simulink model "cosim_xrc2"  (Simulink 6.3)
settings: Solver=ode45  StartTime=0.0  StopTime=10.0  RelTol=1e-3
undefined symbols (not defined in the file or in its folder): netlist
libraries: xbsIndex_r4 x8, adlibrary2 x1, adcosim_example_lib x1

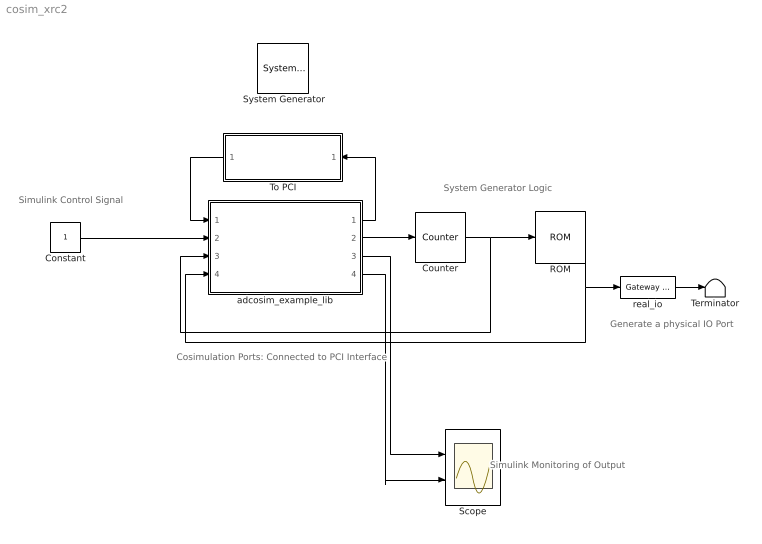
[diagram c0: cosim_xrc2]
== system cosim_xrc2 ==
  note: System Generator Logic
  note: Simulink Control Signal
  note: Simulink Monitoring of Output
  note: Generate a physical IO Port
  note: Cosimulation Ports: Connected to PCI Interface
  " System Generator" : xbsIndex_r4/ System Generator  Tag=genX  xilinxfamily=Virtex2  part=xc2v4000  speed=-4  package=ff1152  synthesis_tool=XST  directory=./netlist  testbench=off  simulink_period=1  sysclk_period=10  incr_netlist=off  trim_vbits=Everywhere in SubSystem  dbl_ovrd=According to Block Masks  core_generation=According to Block Masks  run_coregen=off  deprecated_control=off  eval_field=0  block_type=sysgen
  Constant : Constant
  Counter : xbsIndex_r4/Counter  cnt_type=Free Running  cnt_to=Inf  operation=Up  start_count=0  cnt_by_val=1  arith_type=Unsigned  n_bits=8  bin_pt=0  load_pin=off  rst=off  en=on  dbl_ovrd=off  explicit_period=on  period=1  use_behavioral_HDL=off  use_rpm=off  block_type=counter
  ROM : xbsIndex_r4/ROM  depth=256  initVector=32767*sin(2*pi*(0:255)/256)  distributed_mem=Block RAM  rst=off  init_reg=0  en=off  latency=1  arith_type="Signed  (2's comp)"  n_bits=16  bin_pt=0  dbl_ovrd=off  use_rpm=on  block_type=sprom
  Scope : Scope  NumInputPorts=2
  Terminator : Terminator
  To PCI : Subsystem  Orientation=left
  adcosim_example_lib : Subsystem  Tag=configX  BlockChoice=adcosim_example_lib_sim
  real_io : xbsIndex_r4/Gateway Out  hdl_port=on  timing_constraint=None  locs_specified=on  LOCs={'B3','C2','C9','D9','B5','B4','E9','E8','C6','D6','B10','B9','J10','H11','D11','D10'}  block_type=gatewayout
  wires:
  Counter/1 -> ROM/1, adcosim_example_lib/3(count_sg)
  adcosim_example_lib/1(debug_out) -> To PCI/1(debug_out)
  To PCI/1(debug_in) -> adcosim_example_lib/1(debug_in)
  adcosim_example_lib/2(enable_sg) -> Counter/1
  ROM/1 -> adcosim_example_lib/4(sine_sg), real_io/1
  Constant/1 -> adcosim_example_lib/2(enable_sl)
  adcosim_example_lib/3(count_sl) -> Scope/1
  adcosim_example_lib/4(sine_sl) -> Scope/2
  real_io/1 -> Terminator/1

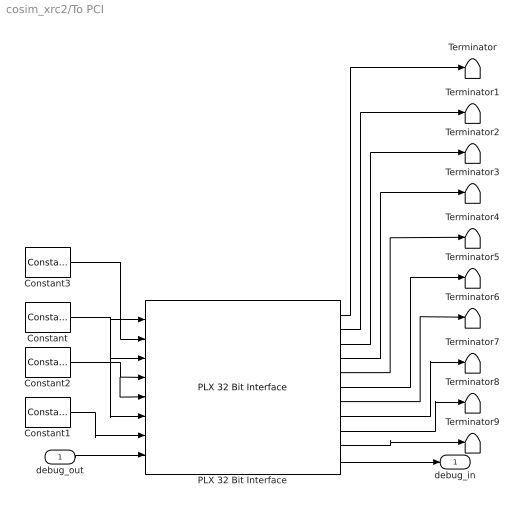
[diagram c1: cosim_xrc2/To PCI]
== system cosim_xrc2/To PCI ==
  debug_out : Inport
  Constant : xbsIndex_r4/Constant  arith_type=Unsigned  const=0  n_bits=32  bin_pt=0  explicit_period=on  period=1  equ=P=C  opselect=C  inp2=PCIN>>17  opr=+  inp1=P  carry=CIN  dbl_ovrd=off  block_type=constant
  Constant1 : xbsIndex_r4/Constant  arith_type=Unsigned  const=0  n_bits=34  bin_pt=0  explicit_period=on  period=1  equ=P=C  opselect=C  inp2=PCIN>>17  opr=+  inp1=P  carry=CIN  dbl_ovrd=off  block_type=constant
  Constant2 : xbsIndex_r4/Constant  arith_type=Boolean  const=0  n_bits=1  bin_pt=0  explicit_period=on  period=1  equ=P=C  opselect=C  inp2=PCIN>>17  opr=+  inp1=P  carry=CIN  dbl_ovrd=off  block_type=constant
  Constant3 : xbsIndex_r4/Constant  arith_type=Boolean  const=1  n_bits=1  bin_pt=0  explicit_period=on  period=1  equ=P=C  opselect=C  inp2=PCIN>>17  opr=+  inp1=P  carry=CIN  dbl_ovrd=off  block_type=constant
  PLX 32 Bit Interface : adlibrary2/ADM-XRC-II/PLX 32 Bit Interface  program='load myprogram.txt'  clock_ratio=1.5
  Terminator{,1..9} (10 alike) : Terminator
  debug_in : Outport
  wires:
  PLX 32 Bit Interface/11 -> debug_in/1
  debug_out/1 -> PLX 32 Bit Interface/8
  PLX 32 Bit Interface/10 -> Terminator9/1
  PLX 32 Bit Interface/9 -> Terminator8/1
  PLX 32 Bit Interface/8 -> Terminator7/1
  PLX 32 Bit Interface/7 -> Terminator6/1
  PLX 32 Bit Interface/6 -> Terminator5/1
  PLX 32 Bit Interface/5 -> Terminator4/1
  PLX 32 Bit Interface/4 -> Terminator3/1
  PLX 32 Bit Interface/3 -> Terminator2/1
  PLX 32 Bit Interface/2 -> Terminator1/1
  PLX 32 Bit Interface/1 -> Terminator/1
  Constant/1 -> PLX 32 Bit Interface/1, PLX 32 Bit Interface/6, PLX 32 Bit Interface/3
  Constant1/1 -> PLX 32 Bit Interface/7
  Constant2/1 -> PLX 32 Bit Interface/4, PLX 32 Bit Interface/5
  Constant3/1 -> PLX 32 Bit Interface/2

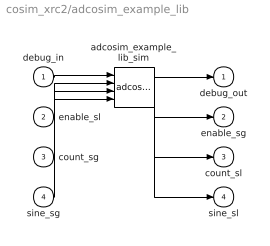
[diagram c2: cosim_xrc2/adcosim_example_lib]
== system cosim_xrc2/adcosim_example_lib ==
  debug_in : Inport
  enable_sl : Inport  Port=2
  count_sg : Inport  Port=3
  sine_sg : Inport  Port=4
  adcosim_example_lib_sim : adcosim_example_lib/adcosim_example_lib_sim
  debug_out : Outport
  enable_sg : Outport  Port=2
  count_sl : Outport  Port=3
  sine_sl : Outport  Port=4
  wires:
  debug_in/1 -> adcosim_example_lib_sim/1
  enable_sl/1 -> adcosim_example_lib_sim/2
  count_sg/1 -> adcosim_example_lib_sim/3
  sine_sg/1 -> adcosim_example_lib_sim/4
  adcosim_example_lib_sim/1 -> debug_out/1
  adcosim_example_lib_sim/2 -> enable_sg/1
  adcosim_example_lib_sim/3 -> count_sl/1
  adcosim_example_lib_sim/4 -> sine_sl/1
